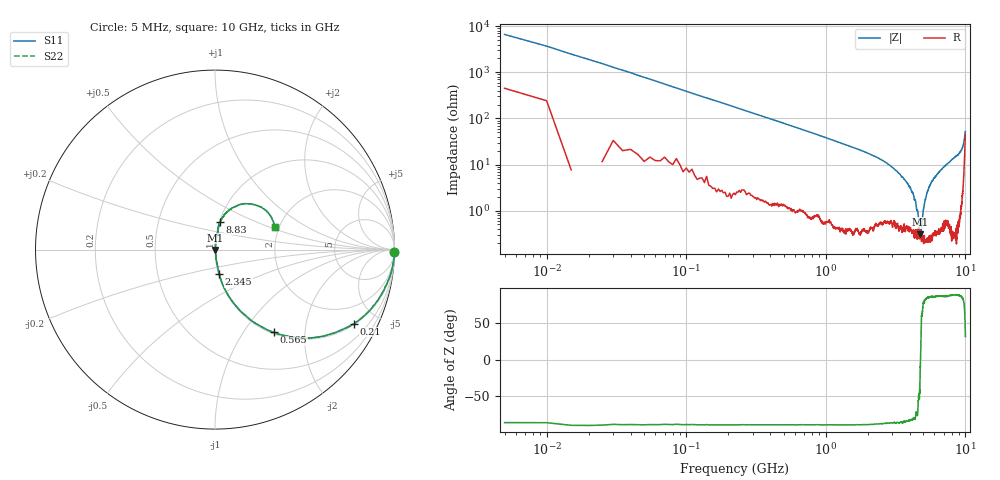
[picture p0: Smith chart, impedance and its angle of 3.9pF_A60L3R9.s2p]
! Amotech Co.,Ltd.
! http://www.amotech.co.kr/
! Part Number: A60L3R9
! These Parameters are Measured in Series Mode Connection
! Operation Temp=25[degC], DC Bias Voltage=0[V]
! Freq. Start=5[MHz] Stop=10[GHz], 2000[Steps]
! Date: Monday, July 14, 2020, 09:31:12
# GHZ S RI R 50.000000
!Freq.(Hz) S11(Real) S11(Imag) S21(Real) S21(Imag) S12(Real) S12(Imag) S22(Real) S22(Imag)
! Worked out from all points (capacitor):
!   2000 points, 5 MHz to 10 GHz, reference 50 ohm
!   read as one part in series: C = 4.1 pF near 55 MHz
!   lowest |Z| = 305 mohm at 4.73 GHz (marker M1)
!   series resonance near 4.77 GHz, so ESL is about 270 pH
!   S11 on the Smith chart (normalised r, x): 5 MHz: open; 210 MHz: 1.04, -3.74; 565 MHz: 1.02, -1.39; 2.345 GHz: 1.01, -0.28; 8.83 GHz: 1.01, +0.32; 10 GHz: 1.89, +0.55
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0.005  0.9987 -0.015  0.00125 0.015  0.00125 0.015  0.9987 -0.015
0.085  0.9484 -0.2069  0.0516 0.2069  0.0516 0.2069  0.9484 -0.2069
0.21  0.7753 -0.4124  0.2247 0.4124  0.2247 0.4124  0.7753 -0.4124
0.355  0.5501 -0.49  0.4499 0.49  0.4499 0.49  0.5501 -0.49
0.565  0.327 -0.4612  0.673 0.4612  0.673 0.4612  0.327 -0.4612
0.975  0.1369 -0.3372  0.8631 0.3372  0.8631 0.3372  0.1369 -0.3372
1.675  0.0489 -0.2065  0.9511 0.2065  0.9511 0.2065  0.0489 -0.2065
2.345  0.0239 -0.1372  0.9761 0.1372  0.9761 0.1372  0.0239 -0.1372
3.34  0.00786 -0.063  0.9921 0.063  0.9921 0.063  0.00786 -0.063
4.22  0.004 -0.0234  0.996 0.0234  0.996 0.0234  0.004 -0.0234
4.565  0.00315 -0.00853  0.9969 0.00853  0.9969 0.00853  0.00315 -0.00853
4.73  0.00273 -0.00134  0.9973 0.00134  0.9973 0.00134  0.00273 -0.00134
4.825  0.00243 0.00275  0.9976 -0.00275  0.9976 -0.00275  0.00243 0.00275
5.005  0.00222 0.0101  0.9978 -0.0101  0.9978 -0.0101  0.00222 0.0101
5.285  0.00271 0.023  0.9973 -0.023  0.9973 -0.023  0.00271 0.023
5.515  0.00375 0.0331  0.9962 -0.0331  0.9962 -0.0331  0.00375 0.0331
6.67  0.0096 0.0745  0.9904 -0.0745  0.9904 -0.0745  0.0096 0.0745
8.335  0.0221 0.1372  0.9779 -0.1372  0.9779 -0.1372  0.0221 0.1372
8.83  0.0292 0.1563  0.9708 -0.1563  0.9708 -0.1563  0.0292 0.1563
9.645  0.0921 0.2288  0.9079 -0.2288  0.9079 -0.2288  0.0921 0.2288
9.865  0.2062 0.2537  0.7938 -0.2537  0.7938 -0.2537  0.2062 0.2537
10  0.3323 0.1272  0.6677 -0.1272  0.6677 -0.1272  0.3323 0.1272
